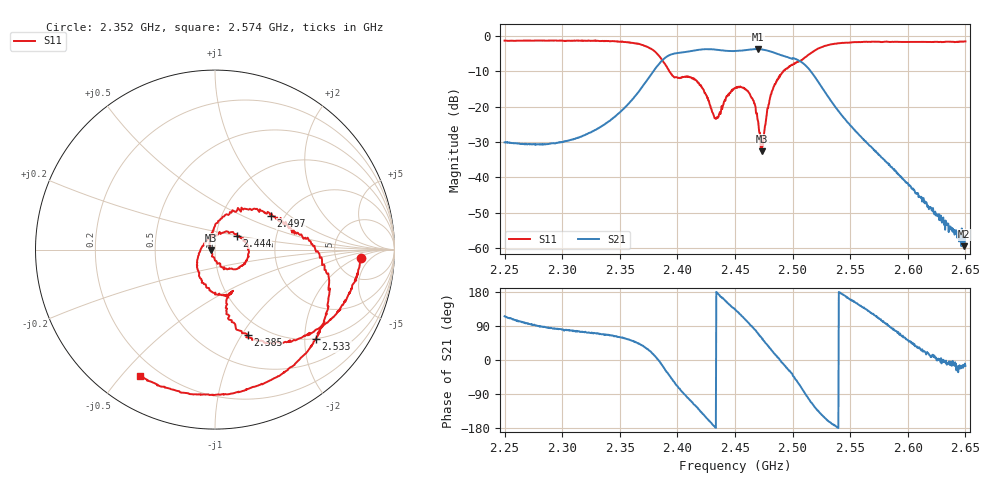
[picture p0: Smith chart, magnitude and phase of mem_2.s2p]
! NanoVNA-App
! Date: 2024-02-22 10:33:23
! Start: 2.25GHz Stop: 2.65GHz Points: 1024
! S-Parameter data: F S11 S21 S12 S22
# Hz S RI R 50
!  Frequency  S11_Real  S11_Imag  S21_Real  S21_Imag  S12_Real  S12_Imag  S22_Real  S22_Imag
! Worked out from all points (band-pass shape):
!   1024 points, 2.25 GHz to 2.65 GHz, reference 50 ohm
!   highest |S21| = -3.81 dB at 2.47 GHz (marker M1); lowest = -59.4 dB at 2.649 GHz (marker M2)
!   |S21| within 3 dB of the highest: 2.387 GHz to 2.504 GHz (116.7 MHz wide, 4.77 % of centre)
!   lowest |S11| = -32.7 dB at 2.473 GHz (marker M3), VSWR 1.05, Z = 47.8 - j0.461 ohm
!   |S11| at or under -10 dB: 2.393 GHz to 2.492 GHz (99.18 MHz wide, 4.06 % of centre)
!   S12 and S22 are empty: the file has one direction only
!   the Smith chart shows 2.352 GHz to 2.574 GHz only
!   S11 on the Smith chart (normalised r, x): 2.352 GHz: 9.16, -2.55; 2.385 GHz: 0.83, -1.06; 2.444 GHz: 1.26, +0.20; 2.497 GHz: 1.70, +0.73; 2.533 GHz: 0.99, -2.27; 2.574 GHz: 0.13, -0.56
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2.25e9  -0.6268 0.5714  -0.0134 0.0282  0 0  0 0
2.282454e9  -0.0493 0.8482  0.00107 0.0296  0 0  0 0
2.316862e9  0.57 0.6266  0.0103 0.0364  0 0  0 0
2.352444e9  0.8148 -0.0465  0.0469 0.0766  0 0  0 0
2.383724e9  0.1927 -0.4902  0.3942 -0.00681  0 0  0 0
2.384506e9  0.1819 -0.4733  0.4071 -0.029  0 0  0 0
2.411095e9  0.0483 -0.252  -0.1686 -0.5762  0 0  0 0
2.433382e9  -0.0531 0.0408  -0.6322 -0.0105  0 0  0 0
2.44433e9  0.1214 0.0777  -0.5188 0.3146  0 0  0 0
2.450196e9  0.1817 0.0246  -0.4164 0.4385  0 0  0 0
2.463099e9  0.0986 -0.109  -0.0335 0.6334  0 0  0 0
2.470137e9  0.000275 -0.0614  0.2267 0.6038  0 0  0 0
2.473265e9  -0.0228 -0.00482  0.3375 0.5406  0 0  0 0
2.482649e9  0.0307 0.1706  0.5403 0.2206  0 0  0 0
2.497116e9  0.3104 0.1874  0.4251 -0.2349  0 0  0 0
2.516667e9  0.5757 -0.0159  -0.1189 -0.2754  0 0  0 0
2.53348e9  0.5634 -0.4984  -0.1159 -0.0278  0 0  0 0
2.573754e9  -0.4158 -0.7059  -0.00812 0.0203  0 0  0 0
2.583529e9  -0.6109 -0.539  -9.48e-06 0.015  0 0  0 0
2.612463e9  -0.8049 0.1246  0.00402 0.00216  0 0  0 0
2.648827e9  -0.3519 0.7433  0.00104 -0.000263  0 0  0 0
2.65e9  -0.3382 0.7533  0.00147 -0.000418  0 0  0 0
